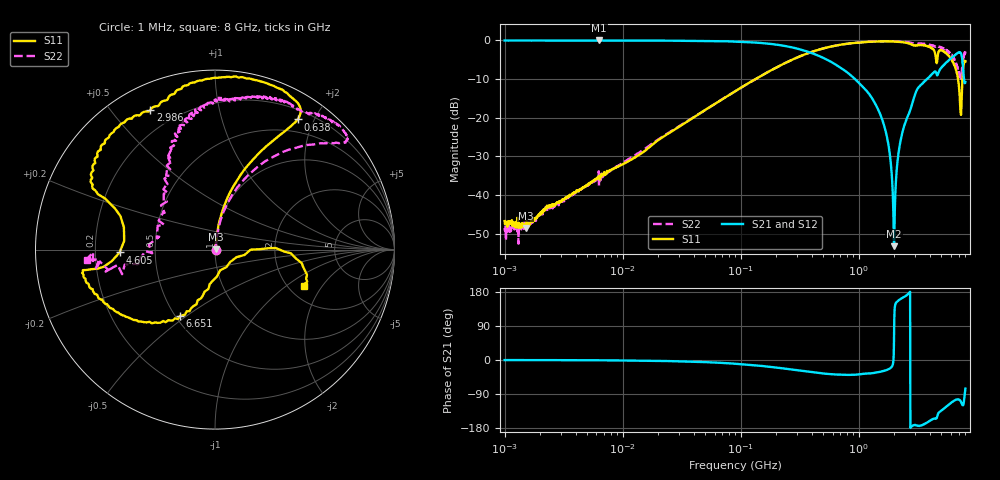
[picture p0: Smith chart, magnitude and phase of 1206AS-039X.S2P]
!s-Parameter Generated by FASTRON Sdn. Bhd.
!FASTRON P/N : 1206AS-039X
!Keysight Technologies: E5071C_MY46733604_B.14.02
!Date: Wed Nov 15 10:10:37 2023
!Version  :Rev00  Wed Nov 15 10:10:37 2023
!Data & Calibration Information:
!Freq  S11:SOLT2(ON)  S21:SOLT2(ON)  S12:SOLT2(ON)  S22:SOLT2(ON)
!PortZ  Port1:50+j0  Port2:50+j0
!When reading reference impedance value at option line is always used.
! Remarks : This data is being provided solely for informational purposes.
# Hz S dB R 50
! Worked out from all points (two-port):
!   1601 points, 1 MHz to 8 GHz, reference 50 ohm
!   highest |S21| = -0.01 dB at 6.301 MHz (marker M1); lowest = -53.2 dB at 1.987 GHz (marker M2)
!   |S21| within 3 dB of the highest: start of sweep to 377.7 MHz
!   lowest |S11| = -48.5 dB at 1.505 MHz (marker M3), VSWR 1.01, Z = 50.3 + j0.181 ohm
!   |S11| at or under -10 dB: start of sweep to 133.2 MHz; 6.929 GHz to 7.556 GHz (627 MHz wide, 8.66 % of centre)
!   |S22| runs from -52.6 to -0.2 dB; largest |S21 - S12| = 0.0078
!   S11 on the Smith chart (normalised r, x): 1 MHz: 1.01, +0.00; 638 MHz: 0.32, +1.77; 2.986 GHz: 0.11, +0.63; 4.605 GHz: 0.31, -0.01; 6.651 GHz: 0.53, -0.47; 8 GHz: 2.43, -1.38
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1000000  -46.71 1.8  -0.03 -0.3  -0.04 -0.2  -48.50 8.2
1504644  -48.52 28.6  -0.03 -0.3  -0.04 -0.2  -48.04 10.2
4479405  -38.23 69.1  -0.04 -0.6  -0.04 -0.6  -38.44 72.5
6301378  -35.46 65.9  -0.01 -1.0  -0.06 -0.8  -37.62 74.4
2.00676e7  -25.73 82.0  -0.06 -2.3  -0.07 -2.3  -25.57 81.4
8.994653e7  -13.08 79.0  -0.30 -9.8  -0.30 -9.8  -13.13 77.0
4.006501e8  -2.96 61.2  -3.28 -32.1  -3.29 -32.1  -2.97 52.4
6.379863e8  -1.32 57.6  -6.26 -38.3  -6.27 -38.3  -1.33 43.7
1.279943e9  -0.31 66.6  -14.71 -34.8  -14.72 -34.9  -0.29 40.1
1.558366e9  -0.26 73.6  -19.98 -30.1  -20.00 -30.3  -0.24 41.5
1.7949e9  -0.27 79.6  -27.50 -24.1  -27.52 -24.3  -0.22 43.5
1.986644e9  -0.31 84.7  -53.19 47.3  -53.35 47.3  -0.23 45.5
2.050559e9  -0.33 86.5  -38.02 148.7  -38.06 148.5  -0.22 45.8
2.125126e9  -0.37 88.5  -31.49 154.7  -31.52 154.5  -0.28 46.1
2.222796e9  -0.41 91.2  -27.07 159.4  -27.09 159.2  -0.33 47.5
2.985754e9  -1.34 114.9  -14.13 -171.3  -14.16 -171.4  -0.82 59.1
4.034495e9  -1.84 146.8  -9.12 -159.3  -9.12 -159.4  -1.19 76.8
4.604562e9  -5.49 -178.3  -9.05 -150.1  -9.04 -150.3  -1.46 86.8
5.220382e9  -2.83 -162.3  -6.48 -129.2  -6.44 -129.4  -2.07 96.1
6.65058e9  -7.59 -117.8  -3.62 -104.7  -3.59 -105.1  -5.67 120.9
7.267458e9  -18.45 -76.5  -3.17 -107.9  -3.15 -108.5  -9.23 157.5
8e9  -5.40 -22.0  -10.79 -75.4  -10.78 -75.9  -2.89 -175.6
